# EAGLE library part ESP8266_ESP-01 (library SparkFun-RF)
ESP8266 ESP-01 Module The ESP8266 WiFi Module is a self contained SOC with integrated TCP/IP protocol stack that can give any microcontroller access to your WiFi network. The ESP8266 is capable of either hosting an application or offloading all Wi-Fi networking functions from another application processor. Each ESP8266 module comes pre-programmed with an AT command set firmware, meaning, you can simply hook this up to your Arduino device and get about as much WiFi-ability as a WiFi Shield offers (and that’s just out of the box)! The ESP8266 module is an extremely cost effective board with a huge, and ever growing, community. This module has a powerful enough on-board processing and storage capability that allows it to be integrated with the sensors and other application specific devices through its GPIOs with minimal development up-front and minimal loading during runtime. Its high degree of on-chip integration allows for minimal external circuitry, including the front-end module, is designed to occupy minimal PCB area. The ESP8266 supports APSD for VoIP applications and Bluetooth co-existance interfaces, it contains a self-calibrated RF allowing it to work under all operating conditions, and requires no external RF parts. SparkFun Product Page
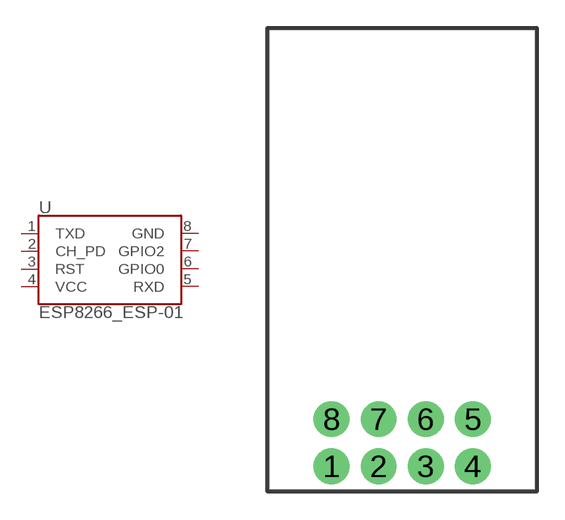
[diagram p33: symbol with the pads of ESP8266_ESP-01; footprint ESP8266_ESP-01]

Designator prefix U

## ESP8266_ESP-01 (SF_ID: WRL-13678)  [ESP8266_ESP-01]
1  TXD
2  CH_PD
3  RST
4  VCC
5  RXD
6  GPIO0
7  GPIO2
8  GND

## Footprint ESP8266_ESP-01 (pad centres in mm)
ESP8266 ESP-01 Module
drill 1.016 pad 1.93: 1 -3.81,-11.13; 2 -1.27,-11.13; 3 1.27,-11.13; 4 3.81,-11.13; 5 3.81,-8.59; 6 1.27,-8.59; 7 -1.27,-8.59; 8 -3.81,-8.59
